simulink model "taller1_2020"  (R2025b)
settings: Solver=VariableStepAuto  StartTime=0.0  StopTime=100  RelTol=1e-3
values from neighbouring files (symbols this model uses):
  a0 = 0.4    [taller_1_tanques.m]
  A2 = 0.5    [taller_1_tanques.m]
  alpha = pi * (R/H)^2    (= 0.223402144255)    [taller_1_tanques.m]
  g = 10    [taller_1_tanques.m]
  h10 = Ho(1)    [taller_1_tanques.m]
  h20 = Ho(2)    [taller_1_tanques.m]
  k0 = 0.25    [taller_1_tanques.m]
  k1 = 0.05    [taller_1_tanques.m]
  k2 = 0.05    [taller_1_tanques.m]
libraries: cstblocks x4, simulink x2

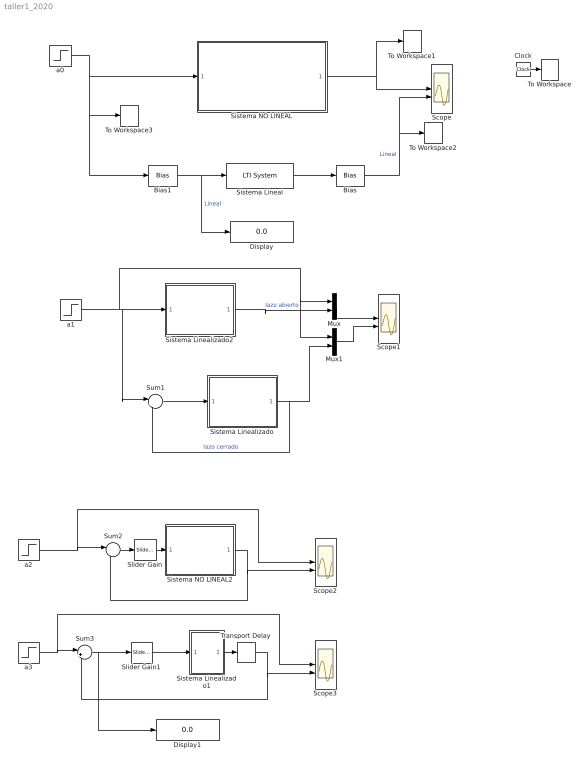
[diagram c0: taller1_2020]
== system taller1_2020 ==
  Bias : Bias  Bias=h20
  Bias1 : Bias  Bias=-a0
  Clock : Clock
  Display : Display
  Display1 : Display
  Mux : Mux  Inputs=2
  Mux1 : Mux  Inputs=2
  Scope{,1..3} (4 alike) : Scope  NumInputPorts=2
  Sistema Lineal : cstblocks/LTI System  sys=G  IC=[]  PadeOrder=0
  Sistema Linealizado : Subsystem
  Sistema Linealizado1 : Subsystem
  Sistema Linealizado2 : Subsystem
  Sistema NO LINEAL : Subsystem
  Sistema NO LINEAL2 : Subsystem
  Slider Gain : simulink/Math Operations/Slider Gain  gain=6.0  low=0  high=6
  Slider Gain1 : simulink/Math Operations/Slider Gain  gain=0.060  low=0  high=6
  Sum1 : Sum  Inputs=|+-
  Sum2 : Sum  Inputs=|+-
  Sum3 : Sum  Inputs=|+-
  To Workspace : ToWorkspace  VariableName=t  SampleTime=-1
  To Workspace1 : ToWorkspace  VariableName=ynl  SampleTime=-1
  To Workspace2 : ToWorkspace  VariableName=yl  SampleTime=-1
  To Workspace3 : ToWorkspace  VariableName=u  SampleTime=-1
  Transport Delay : TransportDelay  DelayTime=10
  a0 : Step  Time=10  Before=a0  After=a0+0.05  SampleTime=0
  a1 : Step  Time=0  Before=a0  After=a0+0.05  SampleTime=0
  a2 : Step  Time=0  Before=a0  After=a0+0.05  SampleTime=0
  a3 : Step  Time=0  After=a0  SampleTime=0
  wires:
  a0/1 -> Bias1/1, To Workspace3/1, Sistema NO LINEAL/1(In1)
  Sistema Lineal/1 -> Bias/1
  Bias/1 -> To Workspace2/1, Scope/2  "Lineal"
  Bias1/1 -> Display/1, Sistema Lineal/1  "Lineal"
  Clock/1 -> To Workspace/1
  Sistema NO LINEAL/1(non-lineal) -> To Workspace1/1, Scope/1
  a1/1 -> Mux1/1, Mux/1, Sistema Linealizado2/1(In1), Sum1/1
  Sum1/1 -> Sistema Linealizado/1(In1)
  Sistema Linealizado/1(Lineal) -> Mux1/2, Sum1/2  "lazo cerrado"
  Mux/1 -> Scope1/1
  Mux1/1 -> Scope1/2
  Sistema NO LINEAL2/1(non-lineal) -> Scope2/2, Sum2/2
  a2/1 -> Sum2/1, Scope2/1
  Sistema Linealizado2/1(Lineal) -> Mux/2  "lazo abierto"
  Sum2/1 -> Slider Gain/1
  Slider Gain/1 -> Sistema NO LINEAL2/1(In1)
  Slider Gain1/1 -> Sistema Linealizado1/1(In1)
  a3/1 -> Scope3/1, Sum3/1
  Sistema Linealizado1/1(Lineal) -> Transport Delay/1
  Transport Delay/1 -> Sum3/2, Scope3/2
  Sum3/1 -> Slider Gain1/1, Display1/1

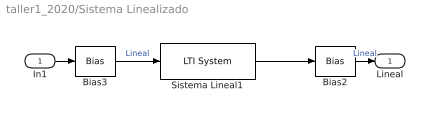
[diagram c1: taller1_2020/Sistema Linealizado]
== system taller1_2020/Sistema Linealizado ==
  In1 : Inport
  Bias2 : Bias  Bias=h20
  Bias3 : Bias  Bias=-a0
  Sistema Lineal1 : cstblocks/LTI System  sys=G  IC=[]  PadeOrder=0
  Lineal : Outport
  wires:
  Bias3/1 -> Sistema Lineal1/1  "Lineal"
  Sistema Lineal1/1 -> Bias2/1
  Bias2/1 -> Lineal/1  "Lineal"
  In1/1 -> Bias3/1

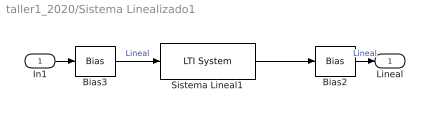
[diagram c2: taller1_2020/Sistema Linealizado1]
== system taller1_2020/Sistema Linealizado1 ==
  In1 : Inport
  Bias2 : Bias  Bias=h20
  Bias3 : Bias  Bias=-a0
  Sistema Lineal1 : cstblocks/LTI System  sys=G  IC=[]  PadeOrder=0
  Lineal : Outport
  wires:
  In1/1 -> Bias3/1
  Bias2/1 -> Lineal/1  "Lineal"
  Sistema Lineal1/1 -> Bias2/1
  Bias3/1 -> Sistema Lineal1/1  "Lineal"

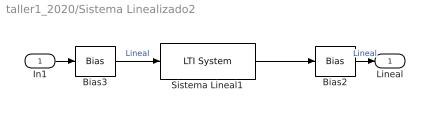
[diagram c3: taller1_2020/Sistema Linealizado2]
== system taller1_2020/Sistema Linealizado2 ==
  In1 : Inport
  Bias2 : Bias  Bias=h20
  Bias3 : Bias  Bias=-a0
  Sistema Lineal1 : cstblocks/LTI System  sys=G  IC=[]  PadeOrder=0
  Lineal : Outport
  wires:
  In1/1 -> Bias3/1
  Bias2/1 -> Lineal/1  "Lineal"
  Sistema Lineal1/1 -> Bias2/1
  Bias3/1 -> Sistema Lineal1/1  "Lineal"

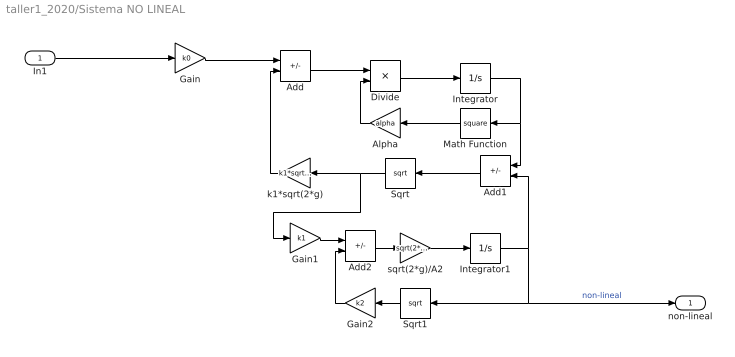
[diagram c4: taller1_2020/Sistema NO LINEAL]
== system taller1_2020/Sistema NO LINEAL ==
  In1 : Inport
  Add : Sum  Inputs=+-
  Add1 : Sum  Inputs=+-
  Add2 : Sum  Inputs=+-
  Alpha : Gain  Gain=alpha
  Divide : Product  Inputs=*/
  Gain : Gain  Gain=k0
  Gain1 : Gain  Gain=k1
  Gain2 : Gain  Gain=k2
  Integrator : Integrator  InitialCondition=h10
  Integrator1 : Integrator  InitialCondition=h20
  Math Function : Math  Operator=square
  Sqrt : Sqrt
  Sqrt1 : Sqrt
  k1*sqrt(2*g) : Gain  Gain=k1*sqrt(2*g)
  sqrt(2*g)/A2 : Gain  Gain=sqrt(2*g)/A2
  non-lineal : Outport
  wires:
  Gain2/1 -> Add2/2
  Sqrt/1 -> Gain1/1, k1*sqrt(2*g)/1
  Add/1 -> Divide/1
  Sqrt1/1 -> Gain2/1
  k1*sqrt(2*g)/1 -> Add/2
  sqrt(2*g)/A2/1 -> Integrator1/1
  Add2/1 -> sqrt(2*g)/A2/1
  Alpha/1 -> Divide/2
  Integrator1/1 -> non-lineal/1, Sqrt1/1, Add1/2  "non-lineal"
  Divide/1 -> Integrator/1
  Gain1/1 -> Add2/1
  Integrator/1 -> Add1/1, Math Function/1
  Gain/1 -> Add/1
  Add1/1 -> Sqrt/1
  Math Function/1 -> Alpha/1
  In1/1 -> Gain/1

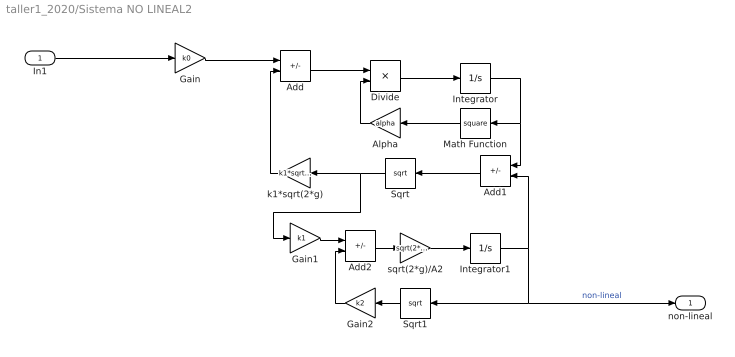
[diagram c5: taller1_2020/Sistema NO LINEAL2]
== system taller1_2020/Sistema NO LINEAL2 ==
  In1 : Inport
  Add : Sum  Inputs=+-
  Add1 : Sum  Inputs=+-
  Add2 : Sum  Inputs=+-
  Alpha : Gain  Gain=alpha
  Divide : Product  Inputs=*/
  Gain : Gain  Gain=k0
  Gain1 : Gain  Gain=k1
  Gain2 : Gain  Gain=k2
  Integrator : Integrator  InitialCondition=h10
  Integrator1 : Integrator  InitialCondition=h20
  Math Function : Math  Operator=square
  Sqrt : Sqrt
  Sqrt1 : Sqrt
  k1*sqrt(2*g) : Gain  Gain=k1*sqrt(2*g)
  sqrt(2*g)/A2 : Gain  Gain=sqrt(2*g)/A2
  non-lineal : Outport
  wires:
  Gain2/1 -> Add2/2
  Sqrt/1 -> Gain1/1, k1*sqrt(2*g)/1
  Add/1 -> Divide/1
  Sqrt1/1 -> Gain2/1
  k1*sqrt(2*g)/1 -> Add/2
  sqrt(2*g)/A2/1 -> Integrator1/1
  Add2/1 -> sqrt(2*g)/A2/1
  Alpha/1 -> Divide/2
  Integrator1/1 -> non-lineal/1, Sqrt1/1, Add1/2  "non-lineal"
  Divide/1 -> Integrator/1
  Gain1/1 -> Add2/1
  Integrator/1 -> Add1/1, Math Function/1
  Gain/1 -> Add/1
  Add1/1 -> Sqrt/1
  Math Function/1 -> Alpha/1
  In1/1 -> Gain/1
